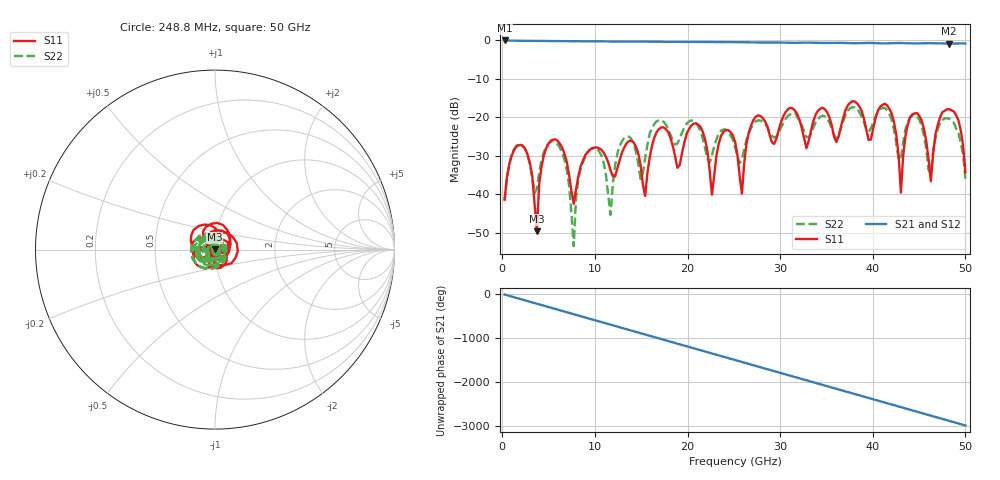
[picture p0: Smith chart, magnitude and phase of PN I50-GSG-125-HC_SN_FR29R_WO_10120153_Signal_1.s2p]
!  2-Port S-parameters as saved by WinCal
!VAR DATE=10-18-2012  09:52:08
!VAR OPNAME=Lynh Bui
# Hz S RI R 50.00
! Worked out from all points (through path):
!   201 points, 248.8 MHz to 50 GHz, reference 50 ohm
!   highest |S21| = -0.04 dB at 248.8 MHz (marker M1); lowest = -0.8 dB at 48.26 GHz (marker M2)
!   group delay of S21, straight-line fit = 166 ps
!   lowest |S11| = -49.7 dB at 3.731 GHz (marker M3), VSWR 1.01, Z = 49.7 + j0.192 ohm
!   |S11| at or under -10 dB: start of sweep to end of sweep
!   |S22| runs from -53.5 to -17.4 dB; largest |S21 - S12| = 0
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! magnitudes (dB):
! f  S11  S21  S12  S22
! 248.8 MHz  -41.4  0.0  0.0  -41.7
! 2.239 GHz  -27.6  -0.1  -0.1  -27.4
! 3.731 GHz  -49.7  -0.2  -0.2  -38.6
! 5.224 GHz  -26.1  -0.2  -0.2  -26.4
! 7.711 GHz  -42.5  -0.2  -0.2  -53.5
! 8.706 GHz  -31.3  -0.3  -0.3  -31.6
! 11.69 GHz  -33.9  -0.3  -0.3  -45.4
! 12.94 GHz  -29.0  -0.3  -0.3  -26.1
! 15.42 GHz  -40.4  -0.4  -0.4  -30.6
! 16.92 GHz  -23.1  -0.4  -0.4  -20.8
! 21.39 GHz  -22.5  -0.4  -0.4  -23.6
! 22.64 GHz  -40.1  -0.4  -0.4  -29.9
! 25.12 GHz  -26.3  -0.5  -0.5  -27.8
! 25.87 GHz  -39.8  -0.5  -0.5  -30.8
! 27.36 GHz  -19.9  -0.6  -0.6  -21.1
! 33.58 GHz  -21.0  -0.6  -0.6  -22.7
! 41.79 GHz  -17.8  -0.8  -0.8  -19.2
! 43.03 GHz  -39.6  -0.7  -0.7  -30.8
! 44.03 GHz  -20.0  -0.8  -0.8  -20.1
! 46.27 GHz  -36.6  -0.8  -0.8  -34.3
! 48.26 GHz  -17.9  -0.8  -0.8  -20.4
! 50 GHz  -34.3  -0.8  -0.8  -36.0
